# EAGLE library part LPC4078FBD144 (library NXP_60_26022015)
32-bit ARM Cortex-M4 MCU; up to 512 kB flash, 96 kB SRAM; USB Device/Host/OTG; Ethernet; LCD; EMC; SPIFI The LPC408x/7x is an ARM Cortex-M4 based digital signal controller for embedded applications requiring a high level of integration and low power dissipation. The ARM Cortex-M4 is a next generation core that offers system enhancements such as low power consumption, enhanced debug features, and a high level of support block integration. The ARM Cortex-M4 CPU incorporates a 3-stage pipeline, uses a Harvard architecture with separate local instruction and data buses as well as a third bus for peripherals, and includes an internal prefetch unit that supports speculative branching. The ARM Cortex-M4 supports single-cycle digital signal processing and SIMD instructions. A hardware floating-point processor is integrated in the core for several versions of the part. The LPC408x/7x adds a specialized flash memory accelerator to accomplish optimal performance when executing code from flash. The LPC408x/7x is targeted to operate at up to 120 MHz CPU frequency. The peripheral complement of the LPC408x/7x includes up to 512 kB of flash program memory, up to 96 kB of SRAM data memory, up to 4032 byte of EEPROM data memory, External Memory controller (EMC), LCD, Ethernet, USB Device/Host/OTG, an SPI Flash Interface (SPIFI), a General Purpose DMA controller, five UARTs, three SSP controllers, three I 2 C-bus interfaces, a Quadrature Encoder Interface, four general purpose timers, two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
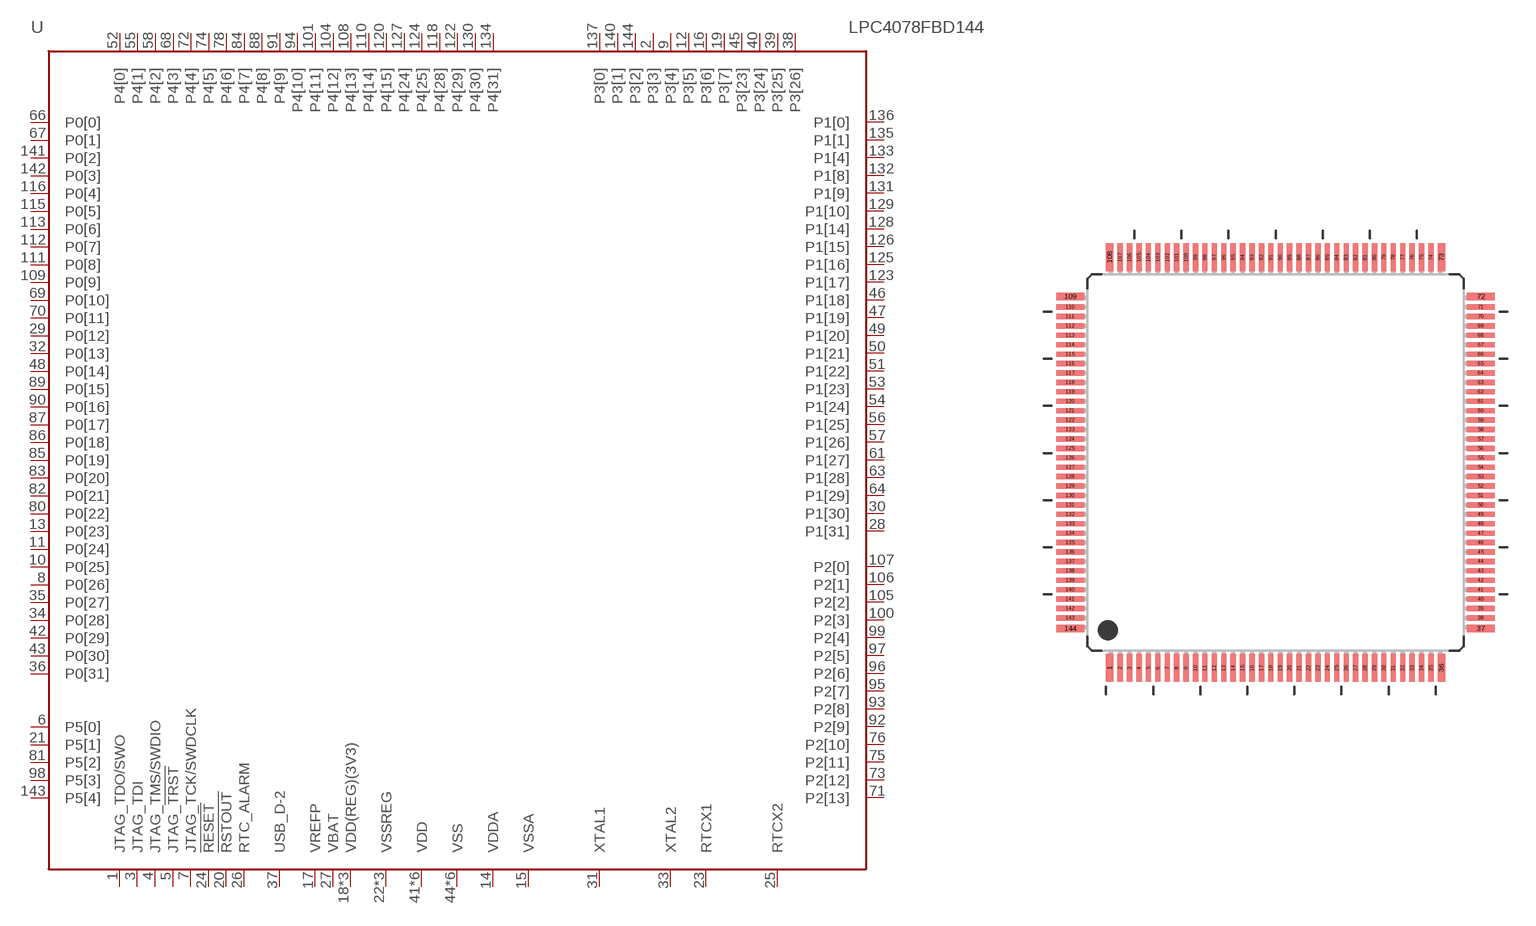
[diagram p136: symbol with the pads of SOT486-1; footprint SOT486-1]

Designator prefix U

## LPC4078FBD144  [SOT486-1]
1  JTAG_TDO/SWO  out
2  P3[3]
3  JTAG_TDI  in
4  JTAG_TMS/SWDIO  in
5  JTAG_!TRST  in
6  P5[0]
7  JTAG_TCK/SWDCLK  in
8  P0[26]
9  P3[4]
10  P0[25]
11  P0[24]
12  P3[5]
13  P0[23]
14  VDDA  pwr
15  VSSA  pwr
16  P3[6]
17  VREFP  pwr
18  VDD(REG)(3V3)  pwr
19  P3[7]
20  !RSTOUT!  out
21  P5[1]
22  VSSREG  pwr
23  RTCX1  in
24  !RESET!  in
25  RTCX2  out
26  RTC_ALARM  out
27  VBAT  pwr
28  P1[31]
29  P0[12]
30  P1[30]
31  XTAL1  in
32  P0[13]
33  XTAL2  out
34  P0[28]
35  P0[27]
36  P0[31]
37  USB_D-2
38  P3[26]
39  P3[25]
40  P3[24]
41  VDD  pwr
42  P0[29]
43  P0[30]
44  VSS  pwr
45  P3[23]
46  P1[18]
47  P1[19]
48  P0[14]
49  P1[20]
50  P1[21]
51  P1[22]
52  P4[0]
53  P1[23]
54  P1[24]
55  P4[1]
56  P1[25]
57  P1[26]
58  P4[2]
59  VSSREG  pwr
60  VDD(REG)(3V3)  pwr
61  P1[27]
62  VDD  pwr
63  P1[28]
64  P1[29]
65  VSS  pwr
66  P0[0]
67  P0[1]
68  P4[3]
69  P0[10]
70  P0[11]
71  P2[13]
72  P4[4]
73  P2[12]
74  P4[5]
75  P2[11]
76  P2[10]
77  VDD  pwr
78  P4[6]
79  VSS  pwr
80  P0[22]
81  P5[2]
82  P0[21]
83  P0[20]
84  P4[7]
85  P0[19]
86  P0[18]
87  P0[17]
88  P4[8]
89  P0[15]
90  P0[16]
91  P4[9]
92  P2[9]
93  P2[8]
94  P4[10]
95  P2[7]
96  P2[6]
97  P2[5]
98  P5[3]
99  P2[4]
100  P2[3]
101  P4[11]
102  VDD  pwr
103  VSS  pwr
104  P4[12]
105  P2[2]
106  P2[1]
107  P2[0]
108  P4[13]
109  P0[9]
110  P4[14]
111  P0[8]
112  P0[7]
113  P0[6]
114  VDD  pwr
115  P0[5]
116  P0[4]
117  VSS  pwr
118  P4[28]
119  VSSREG  pwr
120  P4[15]
121  VDD(REG)(3V3)  pwr
122  P4[29]
123  P1[17]
124  P4[25]
125  P1[16]
126  P1[15]
127  P4[24]
128  P1[14]
129  P1[10]
130  P4[30]
131  P1[9]
132  P1[8]
133  P1[4]
134  P4[31]
135  P1[1]
136  P1[0]
137  P3[0]
138  VDD  pwr
139  VSS  pwr
140  P3[1]
141  P0[2]
142  P0[3]
143  P5[4]
144  P3[2]

## Footprint SOT486-1 (pad centres in mm)
SOT486-1 LQFP144: plastic low profile quad flat package; 144 leads; body 20 x 20 x 1.4 mm JEDEC: MS-026 IEC: 136E23
smd 0.4 x 1.5: 1 -8.81,-10.9; 36 8.81,-10.9; 73 8.81,10.9; 108 -8.81,10.9
smd 0.28 x 1.5: 2 -8.25,-10.9; 3 -7.75,-10.9; 4 -7.25,-10.9; 5 -6.75,-10.9; 6 -6.25,-10.9; 7 -5.75,-10.9; 8 -5.25,-10.9; 9 -4.75,-10.9; 10 -4.25,-10.9; 11 -3.75,-10.9; 12 -3.25,-10.9; 13 -2.75,-10.9; 14 -2.25,-10.9; 15 -1.75,-10.9; 16 -1.25,-10.9; 17 -0.75,-10.9; 18 -0.25,-10.9; 19 0.25,-10.9; 20 0.75,-10.9; 21 1.25,-10.9; 22 1.75,-10.9; 23 2.25,-10.9; 24 2.75,-10.9; 25 3.25,-10.9; 26 3.75,-10.9; 27 4.25,-10.9; 28 4.75,-10.9; 29 5.25,-10.9; 30 5.75,-10.9; 31 6.25,-10.9; 32 6.75,-10.9; 33 7.25,-10.9; 34 7.75,-10.9; 35 8.25,-10.9; 74 8.25,10.9; 75 7.75,10.9; 76 7.25,10.9; 77 6.75,10.9; 78 6.25,10.9; 79 5.75,10.9; 80 5.25,10.9; 81 4.75,10.9; 82 4.25,10.9; 83 3.75,10.9; 84 3.25,10.9; 85 2.75,10.9; 86 2.25,10.9; 87 1.75,10.9; 88 1.25,10.9; 89 0.75,10.9; 90 0.25,10.9; 91 -0.25,10.9; 92 -0.75,10.9; 93 -1.25,10.9; 94 -1.75,10.9; 95 -2.25,10.9; 96 -2.75,10.9; 97 -3.25,10.9; 98 -3.75,10.9; 99 -4.25,10.9; 100 -4.75,10.9; 101 -5.25,10.9; 102 -5.75,10.9; 103 -6.25,10.9; 104 -6.75,10.9; 105 -7.25,10.9; 106 -7.75,10.9; 107 -8.25,10.9
smd 1.5 x 0.4: 37 10.9,-8.81; 72 10.9,8.81; 109 -10.9,8.81; 144 -10.9,-8.81
smd 1.5 x 0.28: 38 10.9,-8.25; 39 10.9,-7.75; 40 10.9,-7.25; 41 10.9,-6.75; 42 10.9,-6.25; 43 10.9,-5.75; 44 10.9,-5.25; 45 10.9,-4.75; 46 10.9,-4.25; 47 10.9,-3.75; 48 10.9,-3.25; 49 10.9,-2.75; 50 10.9,-2.25; 51 10.9,-1.75; 52 10.9,-1.25; 53 10.9,-0.75; 54 10.9,-0.25; 55 10.9,0.25; 56 10.9,0.75; 57 10.9,1.25; 58 10.9,1.75; 59 10.9,2.25; 60 10.9,2.75; 61 10.9,3.25; 62 10.9,3.75; 63 10.9,4.25; 64 10.9,4.75; 65 10.9,5.25; 66 10.9,5.75; 67 10.9,6.25; 68 10.9,6.75; 69 10.9,7.25; 70 10.9,7.75; 71 10.9,8.25; 110 -10.9,8.25; 111 -10.9,7.75; 112 -10.9,7.25; 113 -10.9,6.75; 114 -10.9,6.25; 115 -10.9,5.75; 116 -10.9,5.25; 117 -10.9,4.75; 118 -10.9,4.25; 119 -10.9,3.75; 120 -10.9,3.25; 121 -10.9,2.75; 122 -10.9,2.25; 123 -10.9,1.75; 124 -10.9,1.25; 125 -10.9,0.75; 126 -10.9,0.25; 127 -10.9,-0.25; 128 -10.9,-0.75; 129 -10.9,-1.25; 130 -10.9,-1.75; 131 -10.9,-2.25; 132 -10.9,-2.75; 133 -10.9,-3.25; 134 -10.9,-3.75; 135 -10.9,-4.25; 136 -10.9,-4.75; 137 -10.9,-5.25; 138 -10.9,-5.75; 139 -10.9,-6.25; 140 -10.9,-6.75; 141 -10.9,-7.25; 142 -10.9,-7.75; 143 -10.9,-8.25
